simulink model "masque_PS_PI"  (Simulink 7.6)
settings: Solver=ode45  StartTime=0.0  StopTime=10.0  RelTol=1e-3
libraries: fl_lib x3

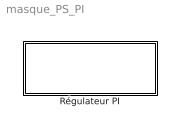
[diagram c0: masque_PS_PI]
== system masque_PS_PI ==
  Régulateur PI : Subsystem  mask(Régulateur PI en composants physiques){K=0}
      mask prompts: K "Gain"

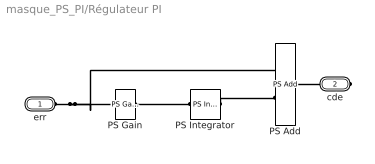
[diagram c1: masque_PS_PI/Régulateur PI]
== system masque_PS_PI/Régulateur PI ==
  PS Add : fl_lib/Physical Signals/Functions/PS Add  DialogController=NetworkEngine.DynNeDlgSource  SystemSampleTime=-1  LocalVarLogging=[]
  PS Gain : fl_lib/Physical Signals/Functions/PS Gain  DialogController=NetworkEngine.DynNeDlgSource  SystemSampleTime=-1  gain=1  LocalVarLogging=[]
  PS Integrator : fl_lib/Physical Signals/Linear Operators/PS Integrator  DialogController=NetworkEngine.DynNeDlgSource  SystemSampleTime=-1  x0=0  x_Log=off  LocalVarNames=|x  LocalVarDescs=|x  LocalVarLogging=0
  err : PMIOPort  Port=1  Side=Left
  cde : PMIOPort  Port=2  Side=Right
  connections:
  err/RConn1 -- PS Add/LConn1 -- PS Gain/LConn1
  PS Integrator/RConn1 -- PS Add/LConn2
  PS Gain/RConn1 -- PS Integrator/LConn1
  cde/RConn1 -- PS Add/RConn1
